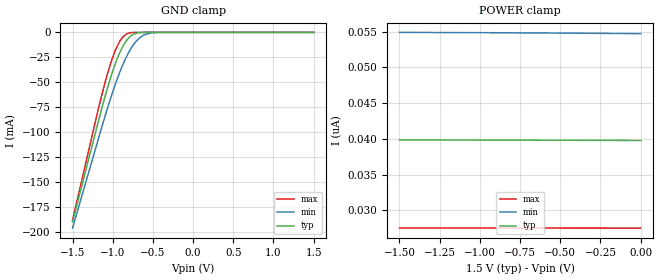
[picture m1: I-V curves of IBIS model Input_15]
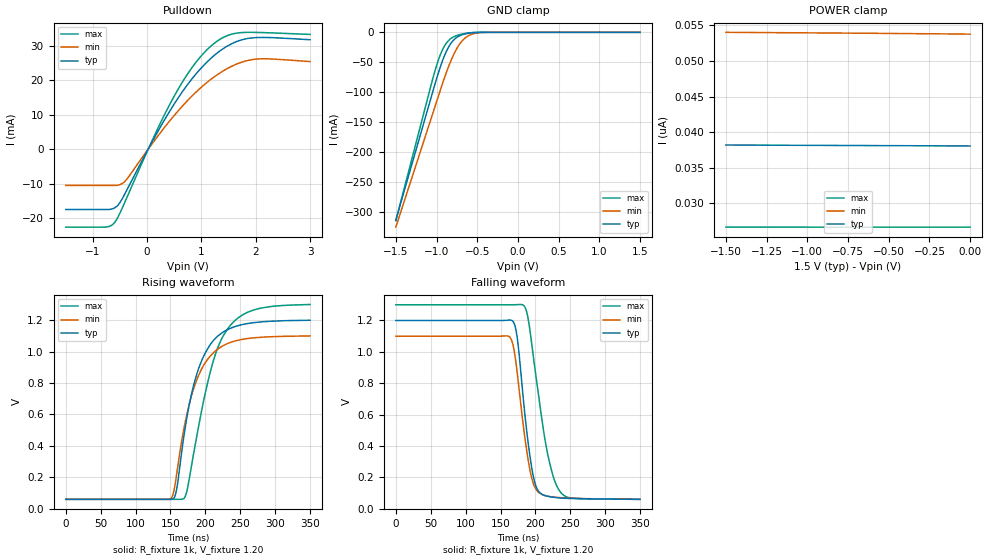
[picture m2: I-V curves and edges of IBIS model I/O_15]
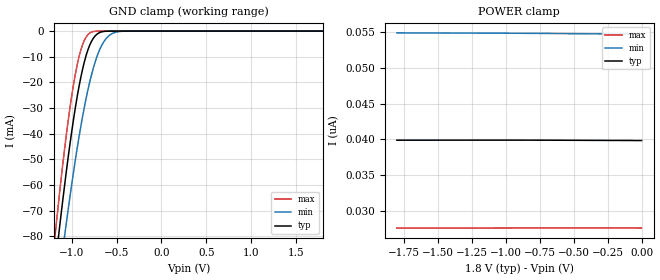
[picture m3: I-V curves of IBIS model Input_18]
|//////////////////////////////////////////////////////////////////////////////
|//////////////////////////////////////////////////////////////////////////////
|   @@@@@@@   @@@@@@@   @@@@@@@   @@@@@@@   @@@@@@@   @@@@@@   @@
|   @@@@@@@@@   @@@@@@@@@   @@@@@@@@@   @@@@@@@@@   @@@@@@@@@ @@@@@@@@  @
|   @@@   @@@ @@@   @@@ @@@   @@@   @@@ @@@   @@@@   @@@  @
|   @@   @@ @@   @@ @@@@@@@@@@@ @@@@@@@@@@@ @@   @@   @@ @@
|   @@@   @@@ @@   @@   @@@ @@@   @@   @@   @@ @@
|   @@@@@@@@@  @@   @@  @@@@@@@@@   @@@@@@@@@  @@   @@   @@ @@
|   @@@@@@@   @@   @@   @@@@@@@   @@@@@@@   @@   @@   @@ @@
|   IBIS Model of N24C008
|   8 Kb I2C CMOS Serial EEPROM in WLCSP-4
|   WLCSP-4  Package Type, CASE 567GG
|   The model is covering the following Vccs:
|   1.5V, 1.8V, 2.2V
|//////////////////////////////////////////////////////////////////////////////
|//////////////////////////////////////////////////////////////////////////////
[IBIS Ver]   3.2
|   7.2 compatible
|//////////////////////////////////////////////////////////////////////////////
[Comment Char] |_char
|//////////////////////////////////////////////////////////////////////////////
[File Name]   n24c008_gb_r0.ibs
|//////////////////////////////////////////////////////////////////////////////
[File Rev]   0.0
|   0.0 - Dec 12, 2024 - File created
|//////////////////////////////////////////////////////////////////////////////
[Date]   Dec 12, 2024
|//////////////////////////////////////////////////////////////////////////////
[Source]   From lab measurements at onsemi
|//////////////////////////////////////////////////////////////////////////////
[Notes]
   - The currents greater than +/- 100 mA are extrapolated
   - The nonmonotonic behavior is expected
|//////////////////////////////////////////////////////////////////////////////
[Disclaimer]
   - onsemi Corporation hereby grants
   the user of this IBIS model a license to use this IBIS
   model under the following terms. This license in nonexclusive
   and nontransferable. Before using this IBIS model.
   After reading the terms and conditions of this license,
   the user either must accept these terms,
   or the IBIS model should be returned to onsemi within 30 days.
   - The user is hereby granted a license to use the IBIS model.
   This shall not be construed as a right to sell,
   or otherwise profit either by leasing or renting this software.
   - The user may modify the IBIS model to suit his specific
   applications but rights to derivative works and such
   modifications shall belong to onsemi.
   - This IBIS model is provided on an "as is" basis.
   onsemi makes absolutely no warranty with respect
   to the information contained herein.
   By use of this IBIS model, the user assumes full risk as to the
   quality and suitablility of the model to his particular use,
   and by using this model assumes the entire risk.
   Under all circumstances the user shall not hold
   onsemi liable in any way for the results obtained.
   onsemi reserves the right to make to improve
   the model for reliability, function, or design.
   onsemi does not convey any license under patent
   rights or any other intellectual property rights,
   including those of third parties.
   - onsemi is not obligated to provide maintenance
   or support for the licensed IBIS model.
   - Cont onsemi at ATTN:LOGIC APPLICATIONS/IBIS MODEL.
   5701 N Pima Rd, Scottsdale, AZ 85250
|//////////////////////////////////////////////////////////////////////////////
[Copyright]   (c) 2024 onsemi Corp.
|//////////////////////////////////////////////////////////////////////////////
|//////////////////////////////////////////////////////////////////////////////
[Component]   N24C008C4DTG
|//////////////////////////////////////////////////////////////////////////////
[Manufacturer]  onsemi
|   Data Sheet: N24C008/D, Rev. 2,  May, 2024
|//////////////////////////////////////////////////////////////////////////////
[Package]
|   WLCSP-4
|  CASE 567GG
| variable   typ   min   max
R_pkg   0.0013   0.0013   0.0013
L_pkg   0.0212nH   0.0212nH   0.0212nH
C_pkg   0.0461pF   0.0461pF   0.0461pF
|//////////////////////////////////////////////////////////////////////////////
[Pin]   signal_name   model_name   R_pin   L_pin   C_pin
1A   VCC   POWER   0.0013   0.0212nH   0.0461pF
2A   GND   GND   0.0013   0.0212nH   0.0461pF
1B   SCL   Input   0.0013   0.0212nH   0.0461pF
2B   SDA   I/O   0.0013   0.0212nH   0.0461pF
|//////////////////////////////////////////////////////////////////////////////
|//////////////////////////////////////////////////////////////////////////////
[Model Selector]   Input
Input_15   Vcc = 1.50
Input_18   Vcc = 1.80
Input_22   Vcc = 2.20
|//////////////////////////////////////////////////////////////////////////////
[Model Selector]   I/O
I/O_15   Vcc = 1.50
I/O_18   Vcc = 1.80
I/O_22   Vcc = 2.20
| Models and submodels in the file (6): Input_15 (Input), I/O_15 (I/O_open_drain), Input_18 (Input), I/O_18 (I/O_open_drain), Input_22 (Input), I/O_22 (I/O_open_drain)
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|//////////////////////////////////////////////////////////////////////////////
|//////////////////////////////////////////////////////////////////////////////
[Model]  Input_15
Model_type Input
Vinh =  0.96
Vinl =  0.24
|  variable   typ   min   max
C_comp   3.8pF   3.8pF   3.8pF
|//////////////////////////////////////////////////////////////////////////////
[Temperature Range]   25   125   -40
|//////////////////////////////////////////////////////////////////////////////
[Voltage Range]   1.50V   1.40V   1.60V
|//////////////////////////////////////////////////////////////////////////////
[POWER Clamp Reference] 1.50V   1.40V   1.60V
|//////////////////////////////////////////////////////////////////////////////
[GND Clamp Reference]   0V   0V   0V
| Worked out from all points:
|   GND clamp passes 1 mA (typ) near -0.71 V on its own axis
|//////////////////////////////////////////////////////////////////////////////
[GND Clamp]
|   Voltage   I(typ)   I(min)   I(max)
-1.5V     -190mA     -196.2mA   -188.4mA
-1.18V    -89.74mA   -107.2mA   -77.3mA
-1.06V    -54.49mA   -74.64mA   -40.15mA
-1V       -38.92mA   -59.63mA   -25.02mA
-940mV    -25.58mA   -45.83mA   -13.25mA
-900mV    -18.13mA   -37.4mA    -7.475mA
-840mV    -9.46mA    -26.28mA   -2.307mA
-760mV    -2.814mA   -14.56mA   -171.9uA
-680mV    -441.6uA   -6.613mA   -6.57uA
-600mV    -31.07uA   -2.292mA   -1.802uA
-520mV    -2.559uA   -545.1uA   -1.33uA
1.5V      39.78nA    54.75nA    27.51nA
|//////////////////////////////////////////////////////////////////////////////
[POWER Clamp]
|   Voltage   I(typ)   I(min)   I(max)
-1.5V     39.86nA    54.91nA    27.54nA
-780mV    39.83nA    54.85nA    27.53nA
-660mV    39.83nA    54.84nA    27.53nA
-600mV    39.82nA    54.83nA    27.52nA
-480mV    39.82nA    54.81nA    27.52nA
-420mV    39.82nA    54.8nA     27.52nA
-360mV    39.81nA    54.79nA    27.52nA
-300mV    39.81nA    54.78nA    27.52nA
-180mV    39.8nA     54.76nA    27.52nA
0V        39.78nA    54.74nA    27.51nA
|//////////////////////////////////////////////////////////////////////////////
|//////////////////////////////////////////////////////////////////////////////
[Model] I/O_15
Model_type I/O_open_drain
Vinh =  0.96
Vinl =  0.24
Vmeas = 0.60
Vref = 1.20
Rref = 1000
Cref = 100pF
|  variable   typ   min   max
C_comp   4.60pF   4.60pF   4.60pF
|//////////////////////////////////////////////////////////////////////////////
[Temperature Range]   25   125   -40
|//////////////////////////////////////////////////////////////////////////////
[Voltage Range]   1.50V   1.40V   1.60V
|//////////////////////////////////////////////////////////////////////////////
[Pulldown Reference]   0V   0V   0V
|//////////////////////////////////////////////////////////////////////////////
[POWER Clamp Reference] 1.50V   1.40V   1.60V
|////////////////////////////////////////////////////////////////////////
[GND Clamp Reference]   0V   0V   0V
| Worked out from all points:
|   slope of the pulldown table from 0 to 0.225 V, typ, clamps not added: 34.8 ohm
|   GND clamp passes 1 mA (typ) near -0.58 V on its own axis
|   falling waveform, R_fixture 1k, V_fixture 1.20: 20-80 % time 16.8ns typ, 18ns min, 24.9ns max; typ from 1.2 V to 0.06 V
|   rising waveform, R_fixture 1k, V_fixture 1.20: 20-80 % time 33.7ns typ, 34.5ns min, 38.8ns max; typ from 0.06 V to 1.2 V
|//////////////////////////////////////////////////////////////////////////////
[Pulldown]
|   Voltage   I(typ)   I(min)   I(max)
-1.5V     -17.52mA   -10.54mA   -22.64mA
-780mV    -17.52mA   -10.54mA   -22.62mA
-620mV    -17.21mA   -10.54mA   -21.67mA
-500mV    -15.48mA   -10.3mA    -18.53mA
-380mV    -12.05mA   -8.813mA   -14.28mA
140mV     3.496mA    2.592mA    4.122mA
500mV     13.11mA    9.777mA    15.4mA
860mV     21.04mA    15.92mA    24.36mA
1.22V     26.96mA    20.77mA    30.48mA
1.5V      30.09mA    23.56mA    33.05mA
1.86V     32.09mA    25.71mA    33.86mA
3V        31.72mA    25.38mA    33.25mA
|//////////////////////////////////////////////////////////////////////////////
[GND Clamp]
|   Voltage   I(typ)   I(min)   I(max)
-1.5V     -313.9mA   -325.6mA   -314.8mA
-1.06V    -105.7mA   -141.3mA   -84.53mA
-1V       -77.77mA   -116.2mA   -55.77mA
-960mV    -60.54mA   -99.43mA   -39.75mA
-920mV    -45.1mA    -82.86mA   -27.27mA
-880mV    -32.07mA   -67.3mA    -18.2mA
-820mV    -17.8mA    -46.45mA   -9.927mA
-740mV    -7.404mA   -24.57mA   -4.87mA
-680mV    -3.742mA   -13.51mA   -2.79mA
-600mV    -1.403mA   -5.163mA   -929.3uA
-500mV    -202.9uA   -1.094mA   -63.25uA
1.5V      38.06nA    53.78nA    26.66nA
|//////////////////////////////////////////////////////////////////////////////
[POWER Clamp]
|   Voltage   I(typ)   I(min)   I(max)
-1.5V     38.19nA    54.01nA    26.67nA
-600mV    38.11nA    53.88nA    26.66nA
-480mV    38.1nA     53.85nA    26.66nA
-300mV    38.08nA    53.82nA    26.66nA
-120mV    38.07nA    53.78nA    26.66nA
-60mV     38.06nA    53.77nA    26.66nA
0V        38.06nA    53.75nA    26.66nA
|//////////////////////////////////////////////////////////////////////////////
|//////////////////////////////////////////////////////////////////////////////
[Ramp]
|  variable   typ   min   max
dV/dt_r   8.280E-01/2.500E-10  0.792E-00/2.500E-10  0.921E+00/2.000E-10
dV/dt_f   0.859E-00/1.800E-08  0.792E-00/1.800E-08  0.921E+00/2.550E-08
R_load = 1k
|//////////////////////////////////////////////////////////////////////////////
|//////////////////////////////////////////////////////////////////////////////
[Falling Waveform]
R_fixture = 1k
V_fixture = 1.20
V_fixture_min = 1.10
V_fixture_max = 1.30
C_fixture = 0p
|   time   V(typ)   V(min)   V(max)
0s        1.2V       1.1V       1.3V
162ns     1.203V     1.099V     1.3V
172.5ns   1.132V     920mV      1.301V
183ns     685.8mV    519.2mV    1.297V
190.5ns   389.9mV    287.1mV    1.188V
201ns     141.2mV    122.7mV    837.8mV
216ns     81.58mV    81.23mV    384.4mV
232.5ns   69.89mV    71.88mV    129.1mV
250.5ns   65.55mV    67.44mV    69.14mV
350ns     60mV       60mV       60mV
|//////////////////////////////////////////////////////////////////////////////
[Rising Waveform]
R_fixture = 1k
V_fixture = 1.20
V_fixture_min = 1.10
V_fixture_max = 1.30
C_fixture = 0p
|   time   V(typ)   V(min)   V(max)
0s        60mV       60mV       60mV
150ns     60.01mV    62.56mV    60mV
157.5ns   93.82mV    177mV      60mV
169.5ns   468.1mV    514.3mV    65.94mV
181.5ns   753.7mV    739.2mV    307mV
193.5ns   928.8mV    878.8mV    597.1mV
211.5ns   1.07V      991.9mV    941.5mV
229.5ns   1.135V     1.047V     1.129V
270ns     1.185V     1.088V     1.266V
350ns     1.2V       1.1V       1.3V
|//////////////////////////////////////////////////////////////////////////////
|//////////////////////////////////////////////////////////////////////////////
[Model]  Input_18
Model_type Input
Vinh =  0.96
Vinl =  0.24
|  variable   typ   min   max
C_comp   3.8pF   3.8pF   3.8pF
|//////////////////////////////////////////////////////////////////////////////
[Temperature Range]   25   125   -40
|//////////////////////////////////////////////////////////////////////////////
[Voltage Range]   1.80V   1.65V   1.95V
|//////////////////////////////////////////////////////////////////////////////
[POWER Clamp Reference] 1.80V   1.65V   1.95V
|//////////////////////////////////////////////////////////////////////////////
[GND Clamp Reference]   0V   0V   0V
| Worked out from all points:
|   GND clamp passes 1 mA (typ) near -0.71 V on its own axis
|//////////////////////////////////////////////////////////////////////////////
[GND Clamp]
|   Voltage   I(typ)   I(min)   I(max)
-1.8V     -285.3mA   -281.7mA   -295.2mA
-1.18V    -89.98mA   -107.4mA   -77.67mA
-1.14V    -77.71mA   -96.17mA   -64.49mA
-1.08V    -60.22mA   -79.94mA   -46.04mA
-1.06V    -54.57mA   -74.7mA    -40.36mA
-980mV    -34.32mA   -54.89mA   -20.78mA
-900mV    -18.19mA   -37.37mA   -7.497mA
-800mV    -5.487mA   -19.9mA    -753uA
-720mV    -1.236mA   -10.02mA   -31.2uA
-660mV    -241.9uA   -5.176mA   -3.749uA
-500mV    -1.721uA   -346.1uA   -1.244uA
1.8V      39.82nA    54.76nA    27.55nA
|//////////////////////////////////////////////////////////////////////////////
[POWER Clamp]
|   Voltage   I(typ)   I(min)   I(max)
-1.8V     39.87nA    54.92nA    27.53nA
-1.14V    39.88nA    54.89nA    27.55nA
-1.02V    39.88nA    54.88nA    27.56nA
-900mV    39.88nA    54.87nA    27.56nA
-840mV    39.88nA    54.86nA    27.56nA
-720mV    39.87nA    54.84nA    27.56nA
-540mV    39.86nA    54.82nA    27.57nA
-360mV    39.85nA    54.79nA    27.56nA
0V        39.82nA    54.74nA    27.56nA
